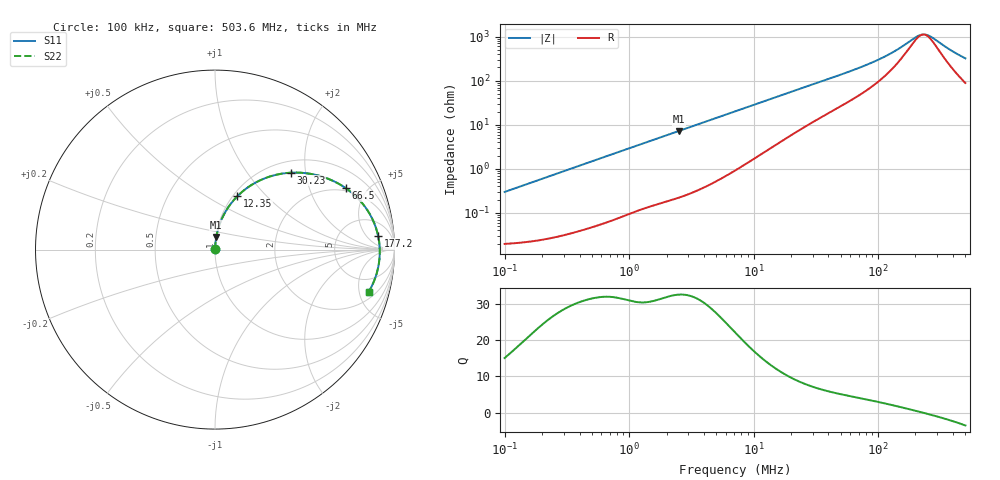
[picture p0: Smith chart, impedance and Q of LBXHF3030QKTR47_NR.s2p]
! LBXHF3030QKTR47_NR  S-PARAMETER MODEL  ( General Type )
! Model Generated by TAIYO YUDEN Corporation (http://www.ty-top.com)
! Version 1.0
! TAIYO YUDEN Control No. 210113NI43SB-FBB
! Copyright(c) 2021 TAIYO YUDEN CO.,LTD. All Rights Reserved.
! Product Description (link to TY-COMPAS)
! https://ds.yuden.co.jp/TYCOMPAS/or/detail?pn=LBXHF3030QKTR47MNR&u=M
! Products Name : Inductors
! Characteristics :
!  Inductance : 0.47 uH , SRF(min) : 150 MHz , DC Resistance(max) : 0.023 Ohm
!  Rated Current : Saturation :3100 mA , Temp Rise : 2200 mA
!  Case Size : 3.0 x 3.0 / 0.118 x 0.118 [mm/inch] , Thickness : 1.5 / 0.059 [mm/inch]
!  (Conditions: Temperature = 25 degC , DC Bias Current/Voltage = 0A / 0V)
! External Node Assignments :
!  1  o---GGG---o  2
! GND o---------o GND
! Frequency Range : 0.1MHz  -  503.601575MHz  [ 402 STEP ]
# MHz S RI R 50
! Freq[MHz].  S11 Real  S11 Imag  S21 Real  S21 Imag  S12 Real  S12 Imag  S22 Real  S22 Imag
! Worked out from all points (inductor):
!   401 points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, 100 kHz to 503.6 MHz, reference 50 ohm
!   read as one part in series: L = 474 nH near 104.4 kHz
!   highest Q = 32.5 at 2.498 MHz (marker M1), where L = 456 nH
!   self-resonance near 231.4 MHz
!   S11 on the Smith chart (normalised r, x): 100 kHz: 1.00, +0.01; 12.35 MHz: 1.05, +0.70; 30.23 MHz: 1.23, +1.66; 66.5 MHz: 1.84, +3.58; 177.2 MHz: 12, +11; 503.6 MHz: 2.77, -6.19
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0.1  0.000206 0.00298  0.9998 -0.00298  0.9998 -0.00298  0.000206 0.00298
0.416965  0.000552 0.0123  0.9994 -0.0123  0.9994 -0.0123  0.000552 0.0123
1.738598  0.00409 0.0498  0.9959 -0.0498  0.9959 -0.0498  0.00409 0.0498
2.497686  0.00726 0.0709  0.9927 -0.0709  0.9927 -0.0709  0.00726 0.0709
4.346839  0.0192 0.1212  0.9808 -0.1212  0.9808 -0.1212  0.0192 0.1212
7.249345  0.0491 0.1943  0.9509 -0.1943  0.9509 -0.1943  0.0491 0.1943
12.35035  0.1253 0.2981  0.8747 -0.2981  0.8747 -0.2981  0.1253 0.2981
18.5152  0.2341 0.3776  0.7659 -0.3776  0.7659 -0.3776  0.2341 0.3776
29.58987  0.4132 0.4279  0.5868 -0.4279  0.5868 -0.4279  0.4132 0.4279
30.22723  0.4221 0.4285  0.5779 -0.4285  0.5779 -0.4285  0.4221 0.4285
44.36007  0.5814 0.411  0.4186 -0.411  0.4186 -0.411  0.5814 0.411
66.50302  0.7279 0.3428  0.2721 -0.3428  0.2721 -0.3428  0.7279 0.3428
93.52439  0.8201 0.2587  0.1799 -0.2587  0.1799 -0.2587  0.8201 0.2587
123.3794  0.8713 0.1816  0.1287 -0.1816  0.1287 -0.1816  0.8713 0.1816
146.3135  0.8927 0.1327  0.1073 -0.1327  0.1073 -0.1327  0.8927 0.1327
177.248  0.9087 0.0773  0.0913 -0.0773  0.0913 -0.0773  0.9087 0.0773
214.7229  0.9169 0.0217  0.0831 -0.0217  0.0831 -0.0217  0.9169 0.0217
228.8991  0.9179 0.00311  0.0821 -0.00311  0.0821 -0.00311  0.9179 0.00311
244.0112  0.9182 -0.0156  0.0818 0.0156  0.0818 0.0156  0.9182 -0.0156
271.4475  0.9167 -0.0469  0.0833 0.0469  0.0833 0.0469  0.9167 -0.0469
398.3636  0.891 -0.1626  0.109 0.1626  0.109 0.1626  0.891 -0.1626
503.6016  0.8565 -0.2356  0.1435 0.2356  0.1435 0.2356  0.8565 -0.2356
